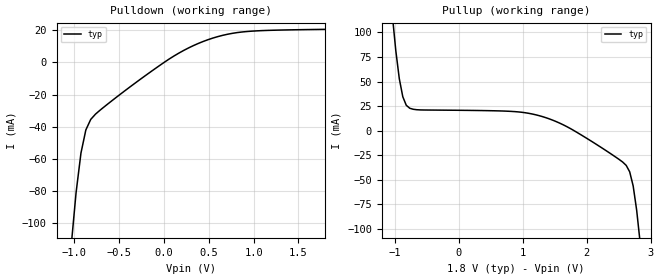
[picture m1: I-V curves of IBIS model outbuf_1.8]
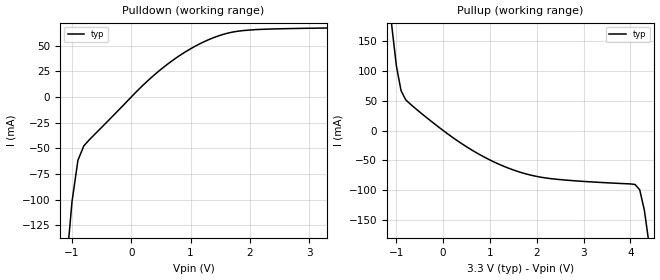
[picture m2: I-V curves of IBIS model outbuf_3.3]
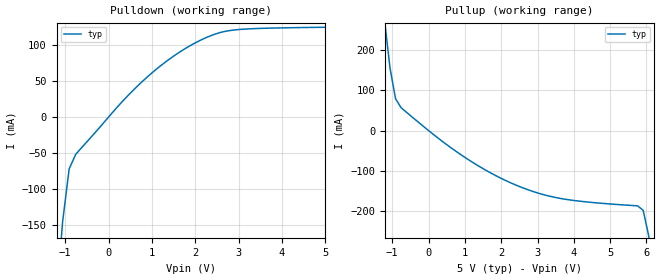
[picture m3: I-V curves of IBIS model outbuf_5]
|Texas Instruments Incorporated
|tmux9616n, 16 Data Lane 1:1 +/-110V Precision mux
[IBIS Ver]   4.1
[File name]   tmux9616n.ibs
[Date]   11/12/24
[File Rev]   1.0
[Source]
| Texas Instruments Incorporated.
| ASC-INT-MPD
| 12500 TI Blvd
| Dallas, TX - 75243
[Notes]   Revision History:
| Rev 1.0: 11/12/24
| - Initial version of the model
| - Model generated from simulations in SPECTRE
| - C_comp although listed in numerical order of value are
|   obtained from varying PVT conditions. For PVT conditions for
|   each specific value refer the buffer description under
|   respective [Model]. IBIS model user is responsible for using
|   appropriate C_comp to simulate for Signal Integrity.
[Disclaimer]
| This model is designed as an aid for customers of Texas Instruments.
| TI and its licensors and suppliers make no warranties, either expressed
| or implied, with respect to this  model, including the warranties of
| merchantability or fitness for a particular purpose. The model is
| provided solely on an "as is" basis. The entire risk as to its quality
| and performance is with the customer.
| This model is subject to change without notice. Texas Instruments
| Incorporated is not responsible for updating this model.
[Copyright]
(C) Copyright 2024 Texas Instruments Incorporated.All rights reserved.
|  Component TMUX9616NPT 48-pin - PT package
|  Part # TMUX9616NPT
[Component]   TMUX9616NPT
[Manufacturer]  TI
[Package]
|   typ   min   max
R_pkg   0.0668   NA   NA
L_pkg   1nH   NA   NA
C_pkg   0.2884pF   NA   NA
[Pin]   signal_name   model_name
   1   nc   nc
   2   nc   nc
   3   D4   dterm
   4   S4   sterm
   5   D3   dterm
   6   S3   sterm
   7   D2   dterm
   8   S2   sterm
   9   D1   dterm
   10   S1   sterm
   11   D0   dterm
   12   S0   sterm
   13   VSS   power
   14   nc   nc
   15   VDD   power
   16   nc   nc
   17   GND   gnd
   18   VLL   power
   19   DIN   inbuf
   20   CLK   inbuf
   21   LE   inbuf_pu
   22   CLR   inbuf
   23   DOUT   outbuf
   24   RGND   gnd
   25   D15   dterm
   26   S15   sterm
   27   D14   dterm
   28   S14   sterm
   29   D13   dterm
   30   S13   sterm
   31   D12   dterm
   32   S12   sterm
   33   D11   dterm
   34   S11   sterm
   35   nc   nc
   36   nc   nc
   37   D10   dterm
   38   S10   sterm
   39   D9   dterm
   40   S9   sterm
   41   D8   dterm
   42   S8   sterm
   43   D7   dterm
   44   S7   sterm
   45   D6   dterm
   46   S6   sterm
   47   D5   dterm
   48   S5   sterm
[Series Switch Groups]
On 1 /
Off 1 /
[Series Pin Mapping]  pin_2 model_name function_table_group
   4   3  switch_dual_110   1
   6   5  switch_dual_110   1
   8   7  switch_dual_110   1
  10   9  switch_dual_110   1
  12  11  switch_dual_110   1
  26  25  switch_dual_110   1
  28  27  switch_dual_110   1
  30  29  switch_dual_110   1
  32  31  switch_dual_110   1
  34  33  switch_dual_110   1
  38  37  switch_dual_110   1
  40  39  switch_dual_110   1
  42  41  switch_dual_110   1
  44  43  switch_dual_110   1
  46  45  switch_dual_110   1
  48  47  switch_dual_110   1
[Model Selector] sterm
sterm_dual_110 Use for operation at +/-110V
[Model Selector] dterm
dterm_dual_110 Use for operation at +/-110V
[Model Selector] inbuf_pu
inbuf_pu_1.8 Use for operation at 1V
inbuf_pu_3.3 Use for operation at 3V
inbuf_pu_5 Use for operation at 5V
[Model Selector] inbuf
inbuf_1.8 Use for operation at 1V
inbuf_3.3 Use for operation at 3V
inbuf_5 Use for operation at 5V
[Model Selector] outbuf
outbuf_1.8 Use for operation at 1V
outbuf_3.3 Use for operation at 3V
outbuf_5 Use for operation at 5V
| switch_dual_110
[Model]   switch_dual_110
Model_type   Series_switch
|   typ   min   max
C_comp   6.362683e-12   NA   NA
[Voltage Range]   110   NA   NA
[Power Clamp Reference]   110   NA   NA
[Temperature Range]   27   NA   NA
[On]
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[Off]
|   typ   min   max
[R Series]   10G   NA   NA
| Models and submodels in the file (12): outbuf_1.8 (Output), outbuf_3.3 (Output), outbuf_5 (Output), inbuf_pu_1.8 (Input), inbuf_pu_3.3 (Input), inbuf_pu_5 (Input), inbuf_1.8 (Input), inbuf_3.3 (Input), inbuf_5 (Input), dterm_dual_110 (Terminator), switch_dual_110 (Series_switch), sterm_dual_110 (Terminator)
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| outbuf_1.8
[Model]   outbuf_1.8
Model_type   Output
|   typ   min   max
C_comp   1.598234e-12   NA   NA
[Voltage Range]   1.8   NA   NA
[Temperature Range]   27   NA   NA
[Pullup Reference]   1.8   NA   NA
[Pulldown Reference]   0   NA   NA
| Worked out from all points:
|   slope of the pulldown table from 0 to 0.27 V, typ, clamps not added: 30.2 ohm
|   slope of the pullup table from 0 to 0.27 V, typ, clamps not added: 1.37 kohm
[Pulldown]
|   Voltage   I(typ)   I(min)   I(max)
-3.6V     -2.691A    NA         NA
-1.036V   -114.4mA   NA         NA
-927.3mV  -56.53mA   NA         NA
-872.7mV  -42.1mA    NA         NA
-818.2mV  -35.54mA   NA         NA
-654.5mV  -27.09mA   NA         NA
54.55mV   2.039mA    NA         NA
272.7mV   9.032mA    NA         NA
490.9mV   14.2mA     NA         NA
709.1mV   17.6mA     NA         NA
927.3mV   19.31mA    NA         NA
1.8V      20.65mA    NA         NA
[Pullup]
|   Voltage   I(typ)   I(min)   I(max)
-1.8V     839.1mA    NA         NA
-1.036V   117.9mA    NA         NA
-927.3mV  52.89mA    NA         NA
-872.7mV  34.5mA     NA         NA
-763.6mV  22.72mA    NA         NA
927.3mV   19.02mA    NA         NA
1.582V    7.457mA    NA         NA
2.618V    -35.54mA   NA         NA
2.673V    -42.1mA    NA         NA
2.727V    -56.53mA   NA         NA
2.836V    -114.4mA   NA         NA
3.6V      -815.1mA   NA         NA
| outbuf_3.3
[Model]   outbuf_3.3
Model_type   Output
|   typ   min   max
C_comp   2.533030e-12   NA   NA
[Voltage Range]   3.3   NA   NA
[Temperature Range]   27   NA   NA
[Pullup Reference]   3.3   NA   NA
[Pulldown Reference]   0   NA   NA
[Power Clamp Reference]   3.3   NA   NA
[GND Clamp Reference]   0   NA   NA
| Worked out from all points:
|   slope of the pulldown table from 0 to 0.495 V, typ, clamps not added: 18.6 ohm
|   slope of the pullup table from 0 to 0.495 V, typ, clamps not added: 18.4 ohm
[Pulldown]
|   Voltage   I(typ)   I(min)   I(max)
-6.6V     -5.932A    NA         NA
-1.1V     -167.9mA   NA         NA
-1V       -102mA     NA         NA
-900mV    -61.7mA    NA         NA
-800mV    -47.6mA    NA         NA
200mV     11.58mA    NA         NA
600mV     31.46mA    NA         NA
900mV     43.49mA    NA         NA
1.2V      53.07mA    NA         NA
1.7V      63.14mA    NA         NA
2.2V      65.9mA     NA         NA
3.3V      67.19mA    NA         NA
[Pullup]
|   Voltage   I(typ)   I(min)   I(max)
-3.3V     2.422A     NA         NA
-1.1V     175.6mA    NA         NA
-1V       107.9mA    NA         NA
-900mV    66.4mA     NA         NA
-800mV    51.2mA     NA         NA
700mV     -36.57mA   NA         NA
1.4V      -62.93mA   NA         NA
2V        -76.6mA    NA         NA
4.1V      -89.98mA   NA         NA
4.2V      -98.85mA   NA         NA
4.4V      -189.5mA   NA         NA
6.6V      -2.38A     NA         NA
| outbuf_5
[Model]   outbuf_5
Model_type   Output
|   typ   min   max
C_comp   2.533030e-12   NA   NA
[Voltage Range]   5   NA   NA
[Temperature Range]   27   NA   NA
[Pullup Reference]   5   NA   NA
[Pulldown Reference]   0   NA   NA
[Power Clamp Reference]   5   NA   NA
[GND Clamp Reference]   0   NA   NA
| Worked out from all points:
|   slope of the pulldown table from 0 to 0.75 V, typ, clamps not added: 15.7 ohm
|   slope of the pullup table from 0 to 0.75 V, typ, clamps not added: 14.7 ohm
[Pulldown]
|   Voltage   I(typ)   I(min)   I(max)
-10V      -11.43A    NA         NA
-1.212V   -262.9mA   NA         NA
-1.061V   -146.3mA   NA         NA
-909.1mV  -72.33mA   NA         NA
-757.6mV  -51.87mA   NA         NA
454.5mV   30.36mA    NA         NA
1.212V    71.97mA    NA         NA
1.667V    91.53mA    NA         NA
1.97V     102.3mA    NA         NA
2.576V    117.7mA    NA         NA
3.182V    122.6mA    NA         NA
5V        125mA      NA         NA
[Pullup]
|   Voltage   I(typ)   I(min)   I(max)
-5V       4.291A     NA         NA
-1.212V   272.8mA    NA         NA
-1.061V   154.1mA    NA         NA
-909.1mV  78.67mA    NA         NA
-757.6mV  56.56mA    NA         NA
1.061V    -69.89mA   NA         NA
2.576V    -140.9mA   NA         NA
3.788V    -170.1mA   NA         NA
5.758V    -186.1mA   NA         NA
5.909V    -197.2mA   NA         NA
6.061V    -259.9mA   NA         NA
10V       -4.239A    NA         NA
